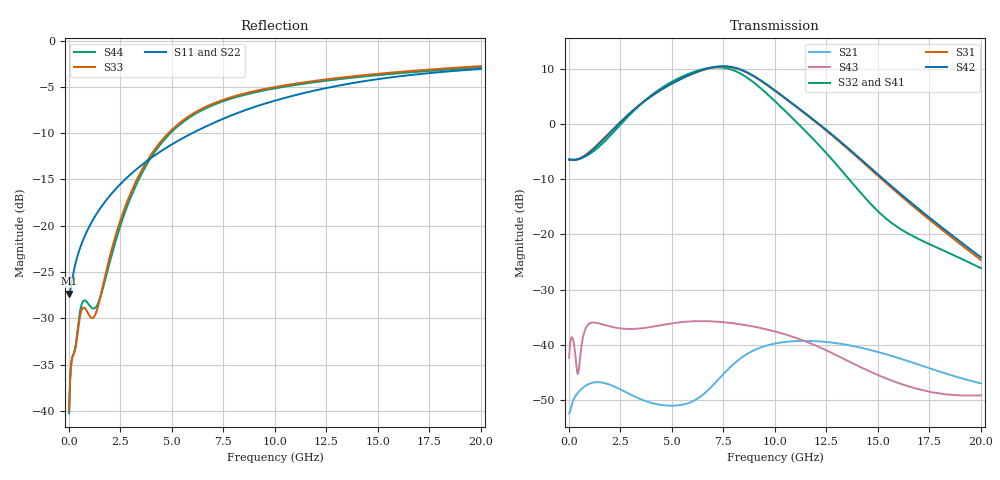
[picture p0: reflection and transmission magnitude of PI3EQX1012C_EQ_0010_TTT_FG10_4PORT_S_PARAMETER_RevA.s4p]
! NPort=4 DATA=2000 NOISE=0 GROUPDELAY=0 COMPLEX_DATAFORMAT=POLAR
! NumOfBlock=1 NumOfParam=0
! .MODEL Smodel S TSTONEFILE=PI3EQX1012C_EQ_0010_TTT_FG10_4PORT_S_PARAMETER_RevA.s4p TYPE=S
!  -- The above .MODEL line can be used for the S element in the netlist.
! The s parameter is extracted from the linear redriver, it is not bi-directional; only s(4,1)s(4,2) and s(3,1)s(3,2)
! should be the insertion loss
!Port definition:
!Port1 = input+
!Port2 = input-
!Port3 = output+
!Port4 = output-
# Hz S MA R  50
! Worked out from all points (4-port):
!   2000 points, 10 MHz to 20 GHz, reference 50 ohm
!   strongest paths, dB at 10 MHz, 5.01 GHz, 10.01 GHz, 15.01 GHz, 20 GHz:
!     S42: -6.4, 7.4, 6.1, -9.1, -24.1
!     S31: -6.4, 7.4, 6.0, -9.4, -24.6
!     S32: -6.4, 7.7, 4.1, -15.8, -26.1
!     S41: -6.4, 7.7, 4.3, -16.0, -26.4
!     S43: -42.4, -36.1, -37.6, -45.5, -49.2
!     S21: -52.4, -51.1, -39.8, -41.3, -47.0
!   lowest |S11| = -27.3 dB at 10 MHz (marker M1), VSWR 1.09, Z = 45.9 - j0.123 ohm
!   |S11| at or under -10 dB: start of sweep to 5.988 GHz
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1e7  0.04301 -178.2  0.002379 1.5  0.0008102 -0.5  0.0008039 -0.5
     0.002388 1.5  0.04109 -178.1  0.000927 -0.5  0.0009197 -0.5
     0.4783 -0.3  0.4774 179.8  0.01016 -4.0  0.007598 -25.7
     0.4769 179.8  0.4792 -0.3  0.007615 -25.8  0.009722 -4.1
5.22e9  0.2843 -123.9  0.002841 16.5  0.0003026 -58.8  0.0003015 -59.6
        0.002809 16.0  0.289 -123.1  0.0003434 -59.7  0.0003422 -60.4
        2.452 -110.6  2.551 82.8  0.3475 -94.6  0.0157 17.8
        2.555 83.1  2.46 -108.7  0.01584 14.6  0.3397 -94.3
7.08e9  0.3614 -124.7  0.004646 44.1  0.0002385 -55.9  0.0002364 -57.2
        0.004467 44.3  0.367 -124.2  0.000269 -57.1  0.0002667 -58.4
        3.287 165.9  3.274 -1.0  0.4603 -109.7  0.01665 -11.2
        3.304 -1.2  3.309 168.1  0.01623 -12.5  0.4522 -109.6
8.34e9  0.4124 -126.1  0.007749 35.8  0.0002217 -54.1  0.0002185 -55.6
        0.007539 36.9  0.4185 -125.7  0.0002483 -55.4  0.0002448 -56.9
        3.108 101.1  2.869 -65.0  0.5113 -117.1  0.01567 -28.2
        2.906 -65.6  3.132 103.6  0.01531 -28.9  0.5028 -117.0
9.89e9  0.4698 -128.5  0.01028 11.8  0.0002115 -54.0  0.0002072 -55.6
        0.01014 12.9  0.4768 -128.1  0.0002351 -55.1  0.0002305 -56.7
        2.08 29.3  1.693 -133.5  0.5579 -123.7  0.01369 -46.4
        1.719 -134.8  2.1 32.1  0.01337 -47.0  0.549 -123.6
1.215e10  0.5437 -132.3  0.0108 -18.8  0.0002008 -57.3  0.0001956 -58.8
          0.01072 -18.0  0.5521 -131.8  0.0002217 -58.0  0.0002164 -59.5
          0.9858 -54.5  0.6422 152.4  0.6098 -130.5  0.00982 -67.8
          0.6492 149.8  1.001 -50.9  0.009522 -68.4  0.6001 -130.4
2e10  0.7023 -144.6  0.004483 -62.6  0.0001466 -72.3  0.0001415 -73.8
      0.004467 -61.5  0.7173 -144.3  0.0001627 -72.1  0.0001569 -73.7
      0.05879 110.3  0.04942 37.4  0.7272 -143.5  0.003559 -51.6
      0.04766 35.4  0.0621 115.0  0.003478 -49.0  0.7152 -143.3
